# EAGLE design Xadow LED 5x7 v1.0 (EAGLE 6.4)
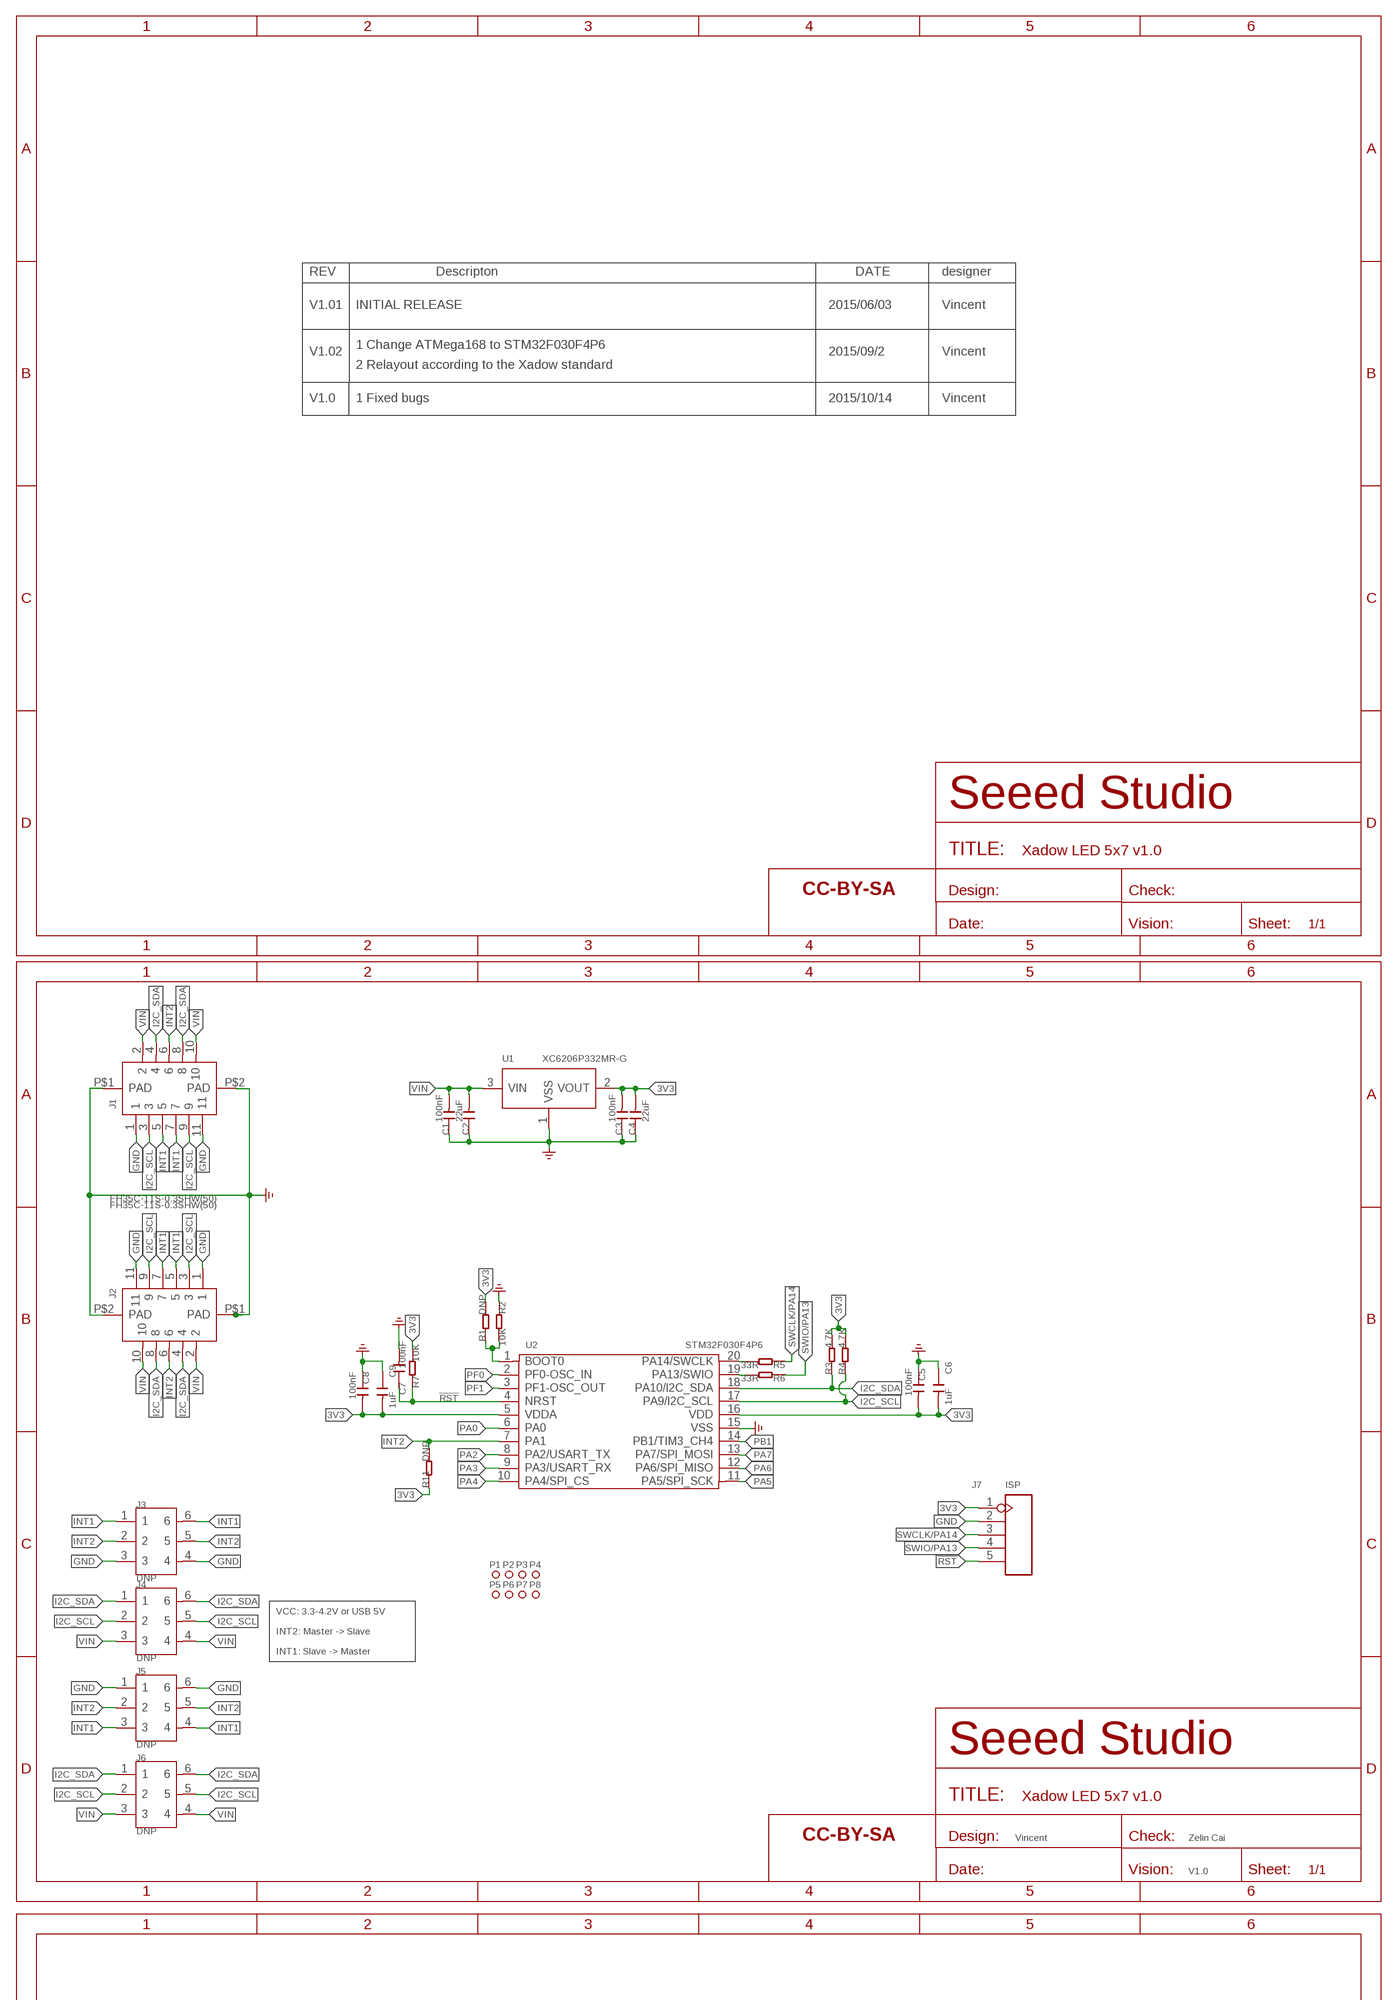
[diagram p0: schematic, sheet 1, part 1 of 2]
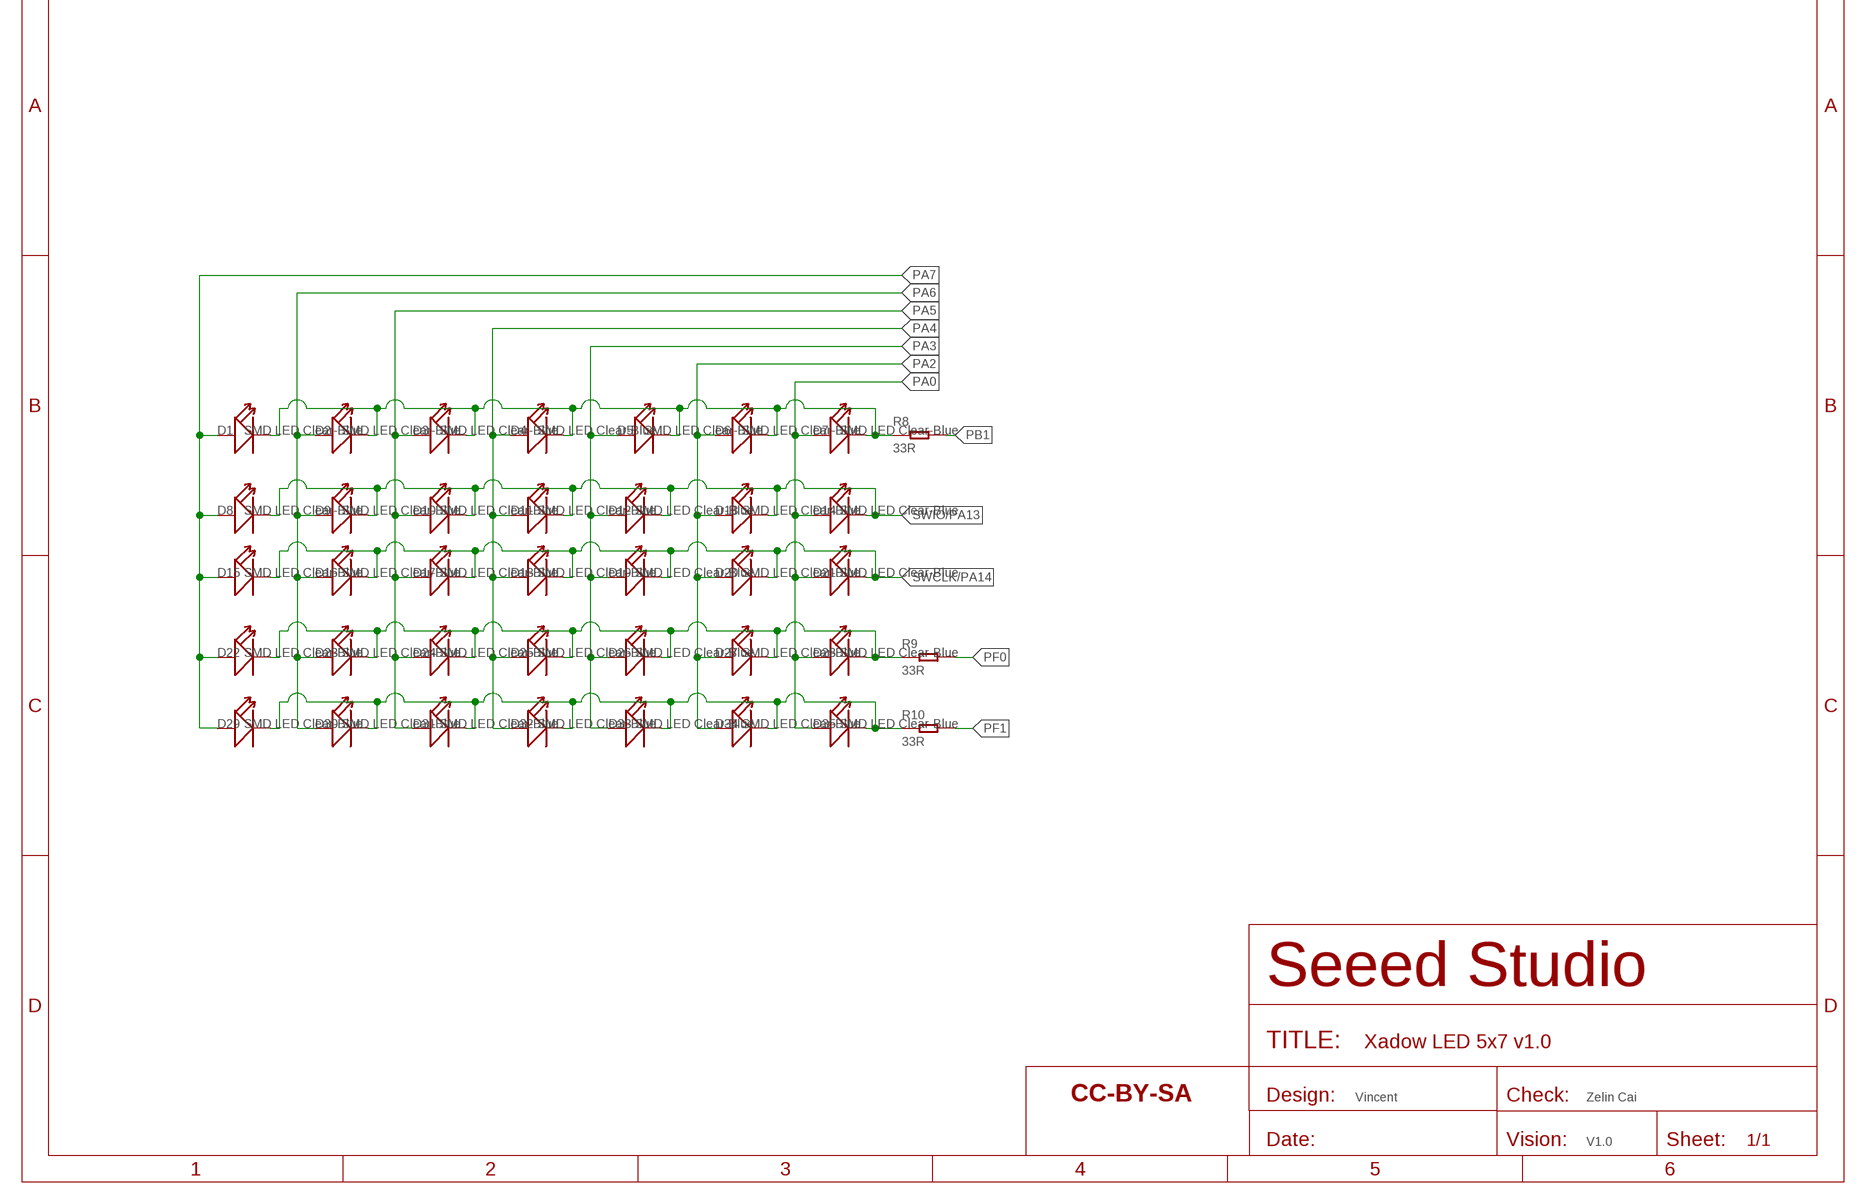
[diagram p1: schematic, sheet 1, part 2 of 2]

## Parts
C1  100nF  CAP-0402  [C0402]
C2  22uF  CAP-0603  [C0603]
C3  100nF  CAP-0402  [C0402]
C4  22uF  CAP-0603  [C0603]
C5  100nF  CAP-0402  [C0402]
C6  1uF  CAP-0402  [C0402]
C7  100nF  CAP-0402  [C0402]
C8  100nF  CAP-0402  [C0402]
C9  1uF  CAP-0402  [C0402]
D1  SMD LED Clear-Blue  LED'0603'  [LED-0603]
D2  SMD LED Clear-Blue  LED'0603'  [LED-0603]
D3  SMD LED Clear-Blue  LED'0603'  [LED-0603]
D4  SMD LED Clear-Blue  LED'0603'  [LED-0603]
D5  SMD LED Clear-Blue  LED'0603'  [LED-0603]
D6  SMD LED Clear-Blue  LED'0603'  [LED-0603]
D7  SMD LED Clear-Blue  LED'0603'  [LED-0603]
D8  SMD LED Clear-Blue  LED'0603'  [LED-0603]
D9  SMD LED Clear-Blue  LED'0603'  [LED-0603]
D10  SMD LED Clear-Blue  LED'0603'  [LED-0603]
D11  SMD LED Clear-Blue  LED'0603'  [LED-0603]
D12  SMD LED Clear-Blue  LED'0603'  [LED-0603]
D13  SMD LED Clear-Blue  LED'0603'  [LED-0603]
D14  SMD LED Clear-Blue  LED'0603'  [LED-0603]
D15  SMD LED Clear-Blue  LED'0603'  [LED-0603]
D16  SMD LED Clear-Blue  LED'0603'  [LED-0603]
D17  SMD LED Clear-Blue  LED'0603'  [LED-0603]
D18  SMD LED Clear-Blue  LED'0603'  [LED-0603]
D19  SMD LED Clear-Blue  LED'0603'  [LED-0603]
D20  SMD LED Clear-Blue  LED'0603'  [LED-0603]
D21  SMD LED Clear-Blue  LED'0603'  [LED-0603]
D22  SMD LED Clear-Blue  LED'0603'  [LED-0603]
D23  SMD LED Clear-Blue  LED'0603'  [LED-0603]
D24  SMD LED Clear-Blue  LED'0603'  [LED-0603]
D25  SMD LED Clear-Blue  LED'0603'  [LED-0603]
D26  SMD LED Clear-Blue  LED'0603'  [LED-0603]
D27  SMD LED Clear-Blue  LED'0603'  [LED-0603]
D28  SMD LED Clear-Blue  LED'0603'  [LED-0603]
D29  SMD LED Clear-Blue  LED'0603'  [LED-0603]
D30  SMD LED Clear-Blue  LED'0603'  [LED-0603]
D31  SMD LED Clear-Blue  LED'0603'  [LED-0603]
D32  SMD LED Clear-Blue  LED'0603'  [LED-0603]
D33  SMD LED Clear-Blue  LED'0603'  [LED-0603]
D34  SMD LED Clear-Blue  LED'0603'  [LED-0603]
D35  SMD LED Clear-Blue  LED'0603'  [LED-0603]
J1  FH35C-11S-0.3SHW(50)  FPC-CONNECTER-11P(FH35C-11S-0.3SHW(50))  [FPC11-SMD-0.3(FH35C)]
J2  FH35C-11S-0.3SHW(50)  FPC-CONNECTER-11P(FH35C-11S-0.3SHW(50))  [FPC11-SMD-0.3(FH35C)]
J3  DNP  HEADER6_ROUND  [6P-DIP-2_ROUND]
J4  DNP  HEADER6  [6P-DIP-2]
J5  DNP  HEADER6_ROUND  [6P-DIP-2_ROUND]
J6  DNP  HEADER6  [6P-DIP-2]
J7  ISP  HEADER-5PTEST  [H5-SMD-2.0-TEST]
P1  MARK-1.0'ANNULAR'  [ROUND-MARK-1.0]
P2  MARK-1.0'ANNULAR'  [ROUND-MARK-1.0]
P3  MARK-1.0'ANNULAR'  [ROUND-MARK-1.0]
P4  MARK-1.0'ANNULAR'  [ROUND-MARK-1.0]
P5  MARK-1.0'ANNULAR'  [ROUND-MARK-1.0]
P6  MARK-1.0'ANNULAR'  [ROUND-MARK-1.0]
P7  MARK-1.0'ANNULAR'  [ROUND-MARK-1.0]
P8  MARK-1.0'ANNULAR'  [ROUND-MARK-1.0]
R1  DNP  RES-0402  [R0402]
R2  10K  RES-0402  [R0402]
R3  4.7K  RES-0402  [R0402]
R4  4.7K  RES-0402  [R0402]
R5  33R  RES-0402  [R0402]
R6  33R  RES-0402  [R0402]
R7  10K  RES-0402  [R0402]
R8  33R  RES-0402  [R0402]
R9  33R  RES-0402  [R0402]
R10  33R  RES-0402  [R0402]
R11  DNP  RES-0402  [R0402]
U1  XC6206P332MR-G  PMIC-XC6206PMR  [SOT-23]
U2  STM32F030F4P6  MCU-STM32F030  [TSSOP20-0.65-6.5X4.4MM]
U$1  SEEEDSTUDIO-OPEN-SCH-FRAME  [SEEEDSTUDIO-PCB-FRAME]
U$2  SEEEDSTUDIO-OPEN-SCH-FRAME  [SEEEDSTUDIO-PCB-FRAME]
U$6  SEEEDSTUDIO-OPEN-SCH-FRAME  [SEEEDSTUDIO-PCB-FRAME]

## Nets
3V3: C3.2 C4.2 C5.2 C6.2 C8.2 C9.2 J7.1 R1.2 R3.2 R4.2 R7.2 R11.1 U1.2(VOUT) U2.5(VDDA) U2.16(VDD)
!RST: C7.1 J7.5 R7.1 U2.4(NRST)
GND: C1.1 C2.1 C3.1 C4.1 C5.1 C6.1 C7.2 C8.1 C9.1 J1.1 J1.11 J1.P$1(PAD) J1.P$2(PAD) J2.1 J2.11 J2.P$1(PAD) J2.P$2(PAD) J3.3 J3.4 J5.1 J5.6 J7.2 R2.1 U1.1(VSS) U2.15(VSS) ; supply symbol labelled GND_POWER
I2C_SCL: J1.3 J1.9 J2.3 J2.9 J4.2 J4.5 J6.2 J6.5 R4.1 U2.17(PA9/I2C_SCL)
I2C_SDA: J1.4 J1.8 J2.4 J2.8 J4.1 J4.6 J6.1 J6.6 R3.1 U2.18(PA10/I2C_SDA)
INT1: J1.5 J1.7 J2.5 J2.7 J3.1 J3.6 J5.3 J5.4
INT2: J1.6 J2.6 J3.2 J3.5 J5.2 J5.5 R11.2 U2.7(PA1)
N$3: D29.- D30.- D31.- D32.- D33.- D34.- D35.- R10.1
N$4: D22.- D23.- D24.- D25.- D26.- D27.- D28.- R9.1
N$5: D1.- D2.- D3.- D4.- D5.- D6.- D7.- R8.1
N$6: R1.1 R2.2 U2.1(BOOT0)
N$7: R5.2 U2.20(PA14/SWCLK)
N$8: R6.2 U2.19(PA13/SWIO)
PA0: D7.+ D14.+ D21.+ D28.+ D35.+ U2.6(PA0)
PA2: D6.+ D13.+ D20.+ D27.+ D34.+ U2.8(PA2/USART_TX)
PA3: D5.+ D12.+ D19.+ D26.+ D33.+ U2.9(PA3/USART_RX)
PA4: D4.+ D11.+ D18.+ D25.+ D32.+ U2.10(PA4/SPI_CS)
PA5: D3.+ D10.+ D17.+ D24.+ D31.+ U2.11(PA5/SPI_SCK)
PA6: D2.+ D9.+ D16.+ D23.+ D30.+ U2.12(PA6/SPI_MISO)
PA7: D1.+ D8.+ D15.+ D22.+ D29.+ U2.13(PA7/SPI_MOSI)
PB1: R8.2 U2.14(PB1/TIM3_CH4)
PF0: R9.2 U2.2(PF0-OSC_IN)
PF1: R10.2 U2.3(PF1-OSC_OUT)
SWCLK/PA14: D15.- D16.- D17.- D18.- D19.- D20.- D21.- J7.3 R5.1
SWIO/PA13: D8.- D9.- D10.- D11.- D12.- D13.- D14.- J7.4 R6.1
VIN: C1.2 C2.2 J1.2 J1.10 J2.2 J2.10 J4.3 J4.4 J6.3 J6.4 U1.3(VIN)

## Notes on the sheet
- REV | Descripton | DATE | designer
- V1.01 | INITIAL RELEASE | 2015/06/03 | Vincent
- 1 Change ATMega168 to STM32F030F4P6
- V1.02 | 2015/09/2 | Vincent
- 2 Relayout according to the Xadow standard
- V1.0 | 1 Fixed bugs | 2015/10/14 | Vincent
- VCC: 3.3-4.2V or USB 5V
- INT2: Master -> Slave
- INT1: Slave -> Master
- Vincent | Zelin Cai
- V1.0
- Vincent | Zelin Cai
- V1.0

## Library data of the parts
C1-C9 = Discrete-new:CAP: Ceramic Capacitors
D1-D35 = Discrete:LED*
J1 J2 = template:FPC-CONNECTER-11P(FH35C-11S-0.3SHW(50))
J3 J5 = template:HEADER6_ROUND
J4 J6 = template:HEADER6
J7 = Connector-new:HEADER-5P
P1-P8 = Discrete-new:MARK-1.0; PARTNO: DNP
R1-R11 = Discrete-new:RES
U1 = IC-new:PMIC-XC6206P: LOW ESR Cap.Compatible Positive Voltage Regulators
U2 = IC-new:MCU-STM32F030
U$1 U$2 U$6 = moudle-new:SEEEDSTUDIO-OPEN-SCH-FRAME

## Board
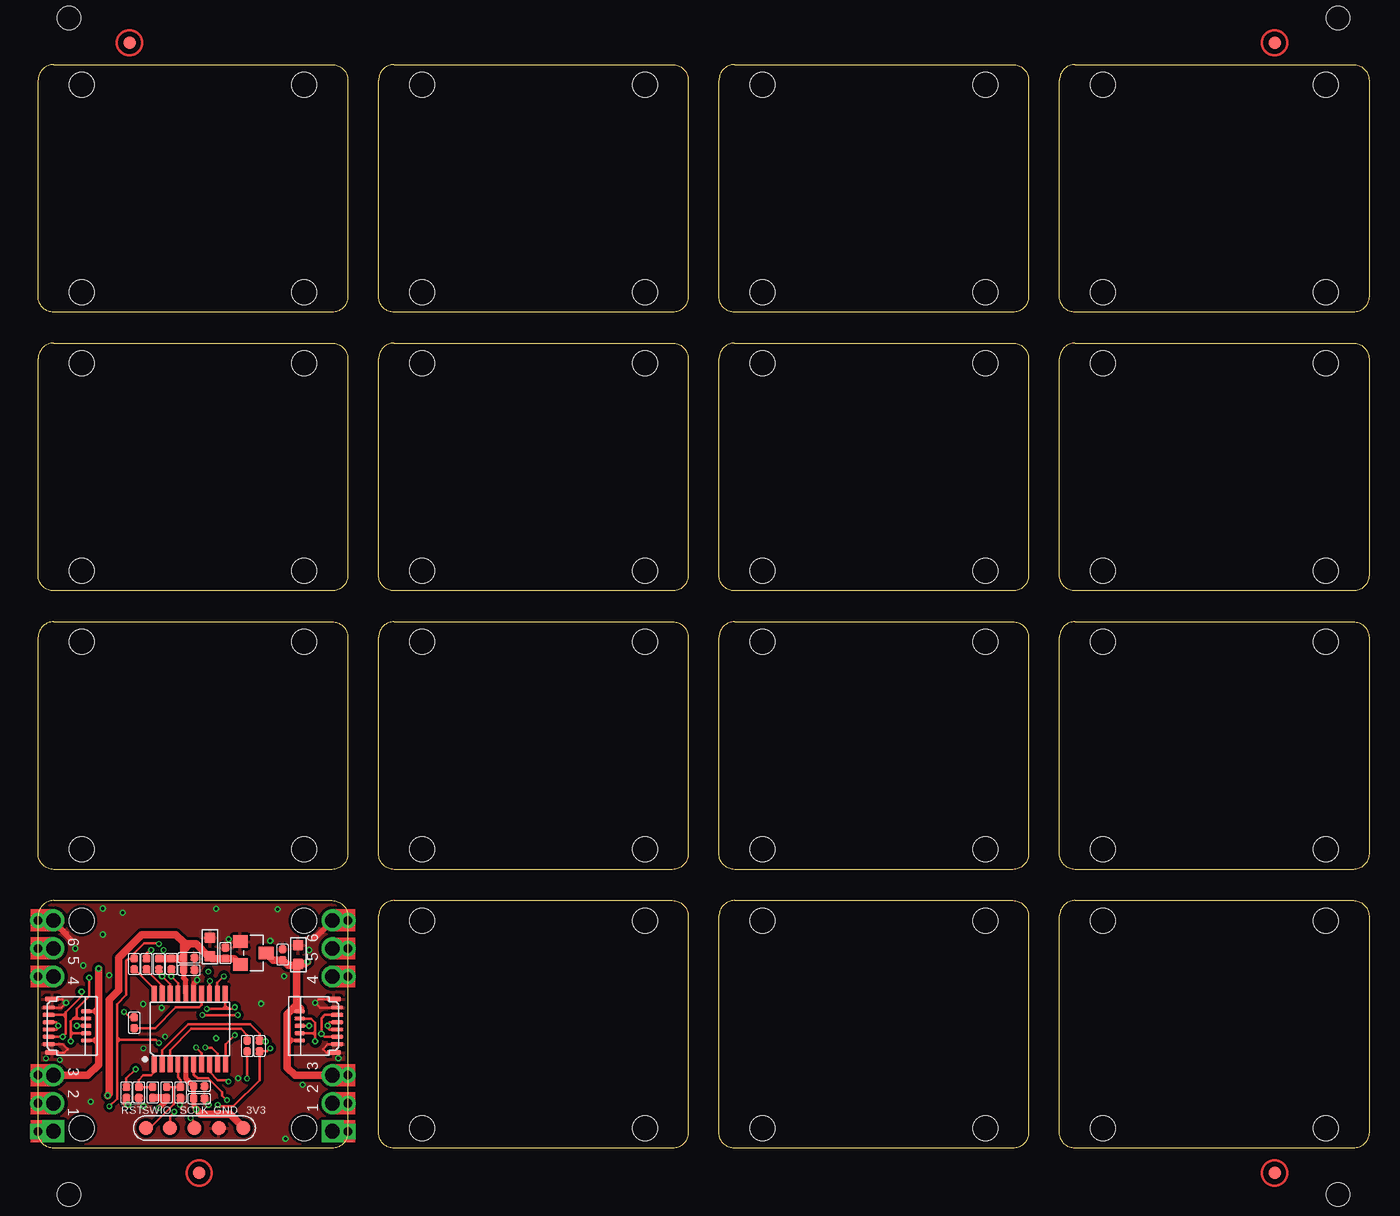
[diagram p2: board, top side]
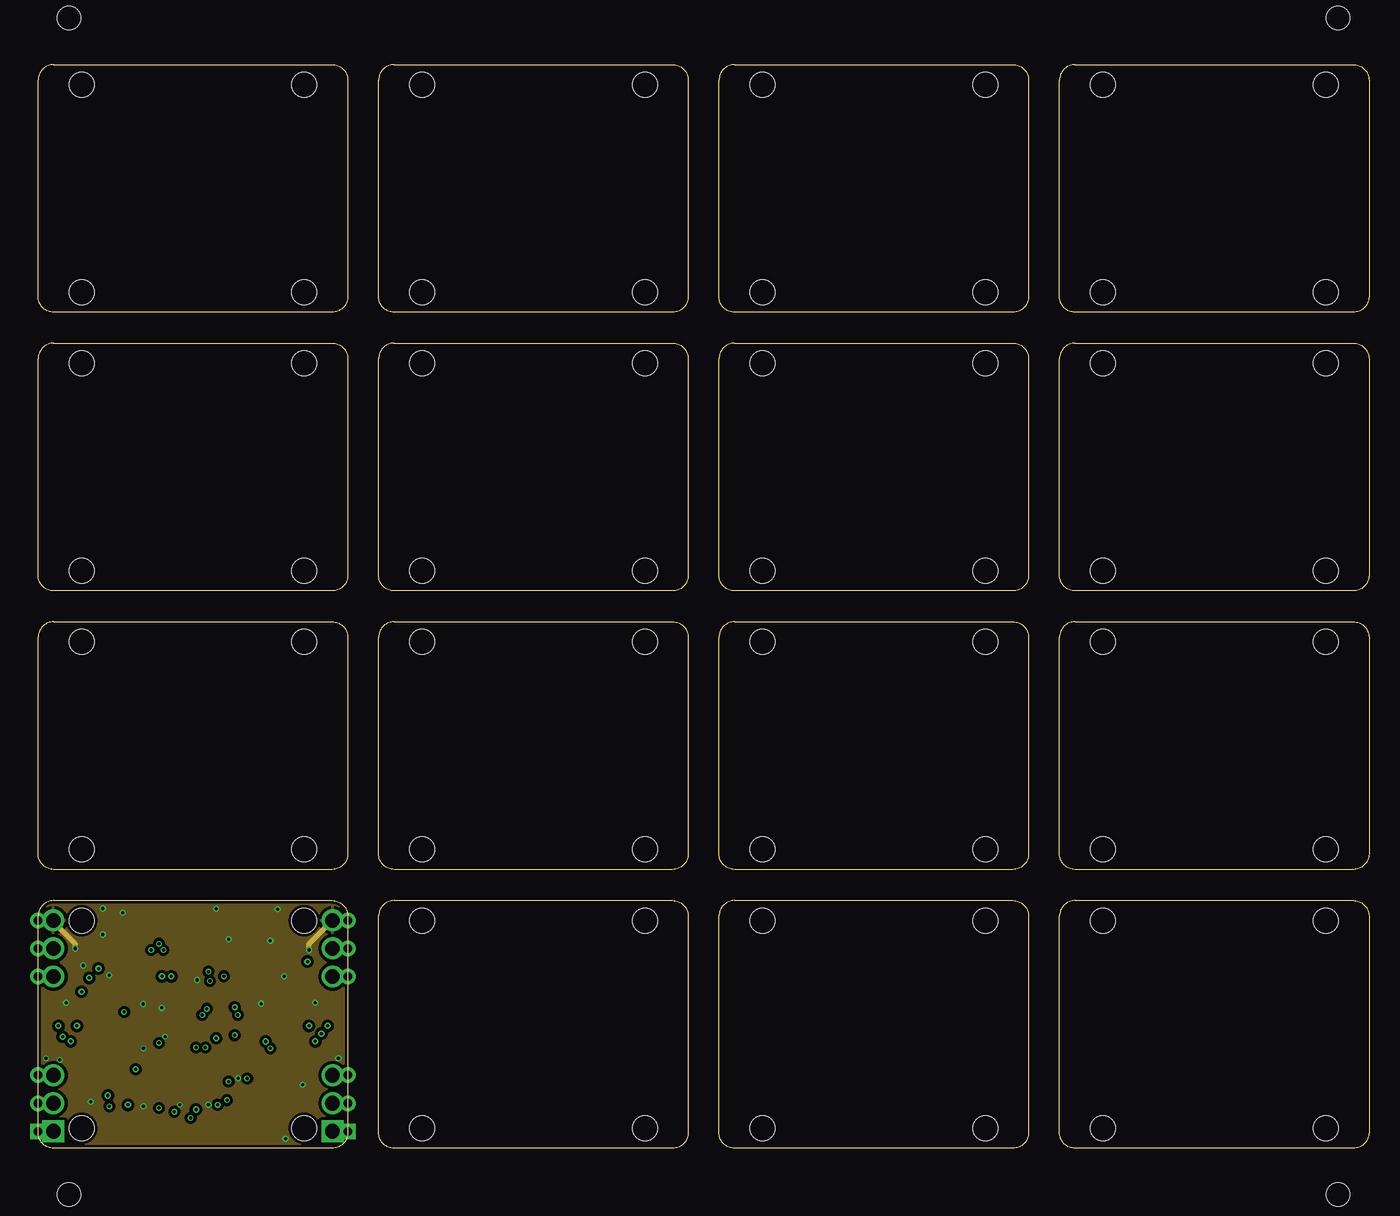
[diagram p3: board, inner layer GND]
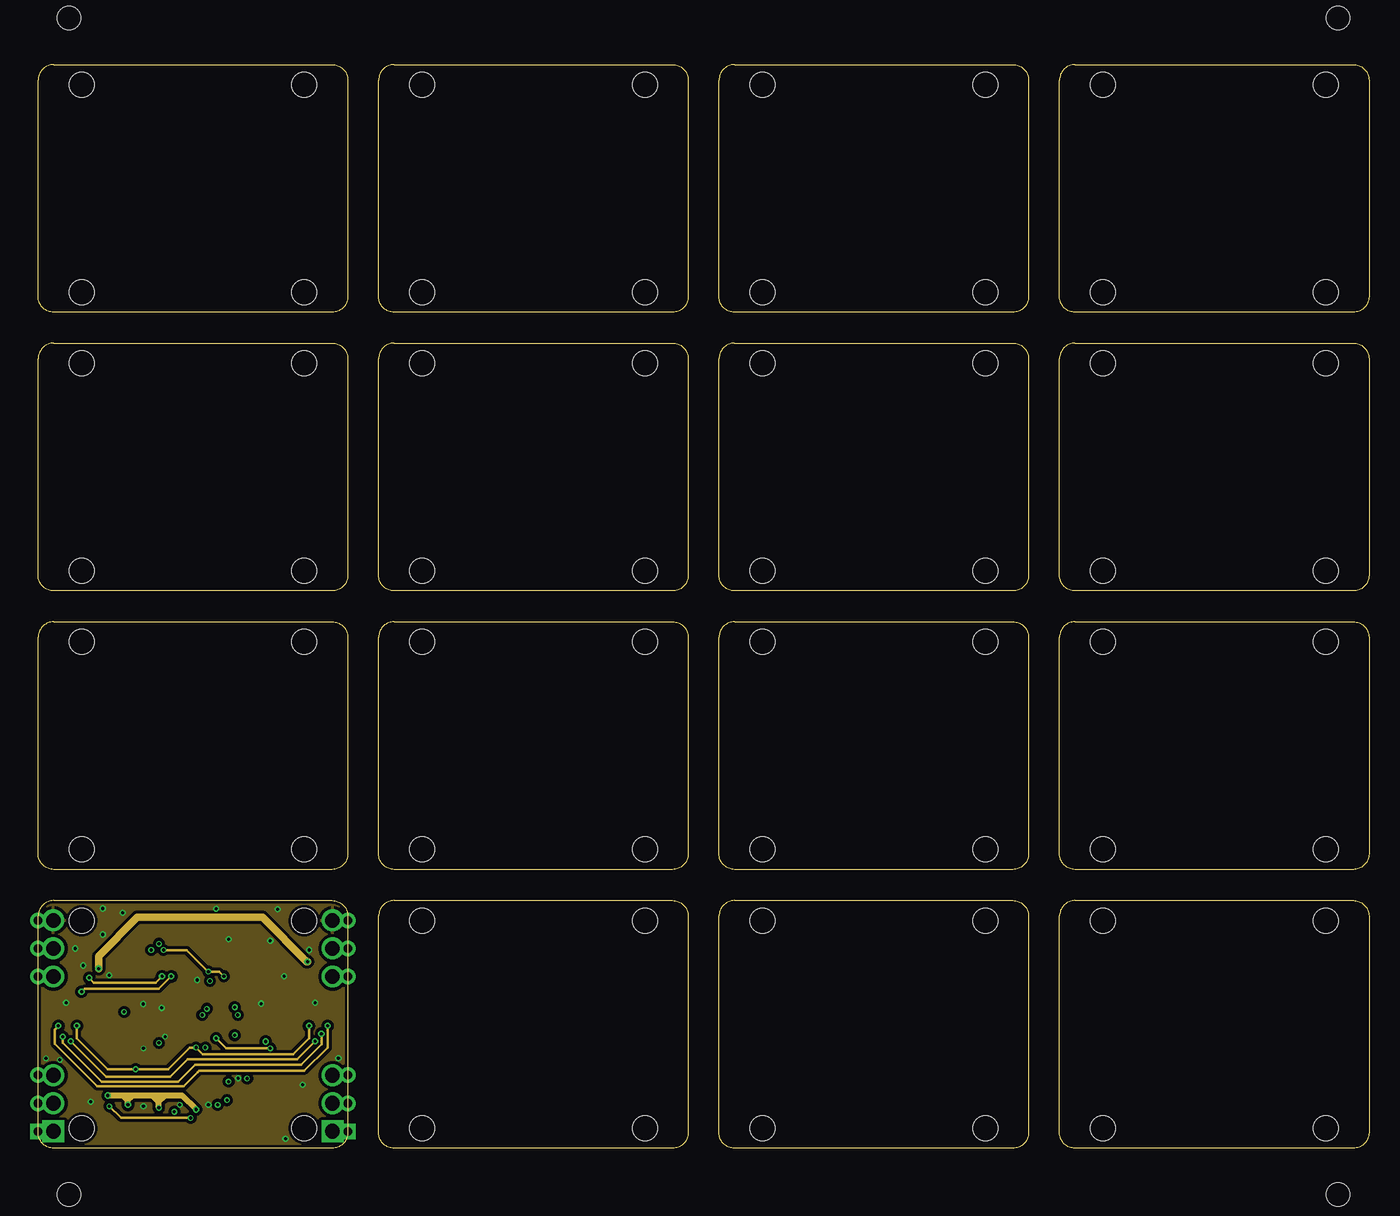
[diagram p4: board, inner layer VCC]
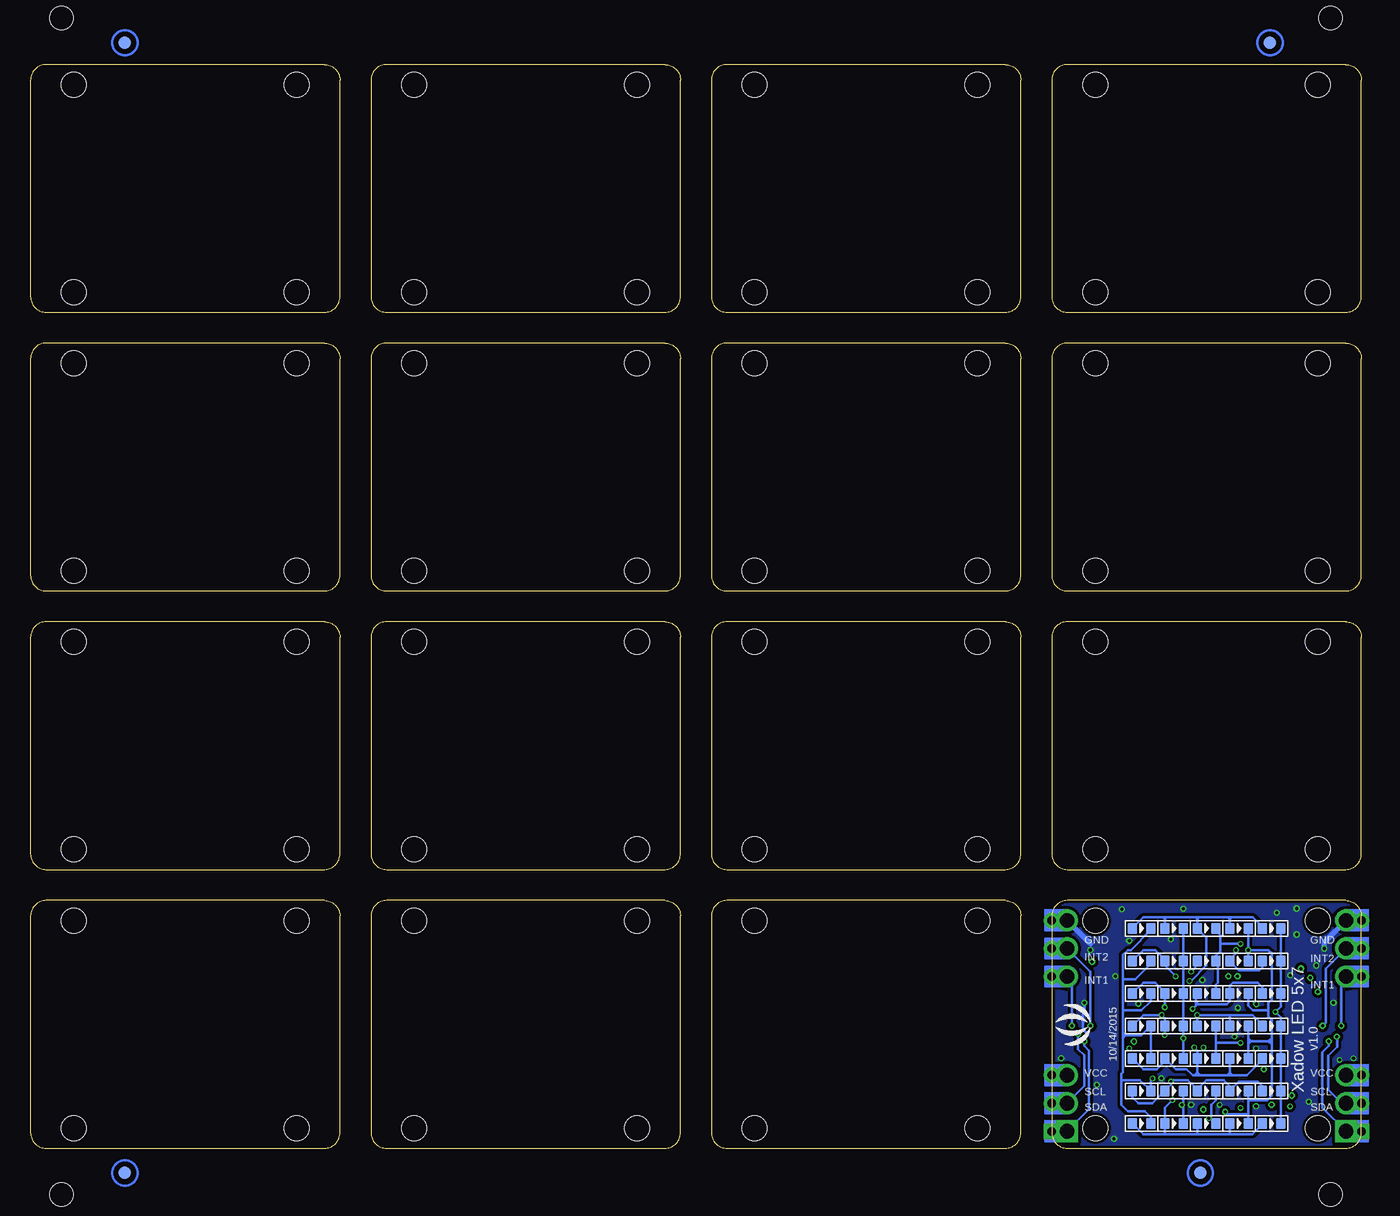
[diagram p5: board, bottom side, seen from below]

Size 109.22 x 88.9 mm. Coordinates in mm from the lower left corner, seen from the top.
Outline: 181 segments
Copper layers (1*2*15*16): Top 0.035mm / dielectric 0.2mm / GND 0.0175mm / dielectric 0.3mm / VCC 0.0175mm / dielectric 0.2mm / Bottom 0.035mm
Design rules "SeeedStudio_4layer_DRU_no_angle_20140221 *": minimum track width 8mil, minimum drill 10mil, track to track 6mil, track to pad 6mil, pad to pad 6mil, via to via 6mil, smd to smd 0mil, copper to edge 10mil, drill to drill 8mil, minimum pad ring 6mil, minimum via ring 4mil, stop-mask expansion 4mil, vias tented up to drill 100mil, thermal gap 10mil
Holes 2.03 mm at 21.84,1.65 21.84,18.67 3.56,18.67 3.56,1.65 3.56,1.65 3.56,18.67 21.84,18.67 21.84,1.65 49.78,1.65 49.78,18.67 31.5,18.67 31.5,1.65 21.84,24.51 21.84,41.53 3.56,41.53 3.56,24.51 49.78,24.51 49.78,41.53 31.5,41.53 31.5,24.51 77.72,1.65 77.72,18.67 59.44,18.67 59.44,1.65 105.66,1.65 105.66,18.67 87.38,18.67 87.38,1.65 77.72,24.51 77.72,41.53 59.44,41.53 59.44,24.51 105.66,24.51 105.66,41.53 87.38,41.53 87.38,24.51 21.84,47.37 21.84,64.39 3.56,64.39 3.56,47.37 49.78,47.37 49.78,64.39 31.5,64.39 31.5,47.37 21.84,70.23 21.84,87.25 3.56,87.25 3.56,70.23 49.78,70.23 49.78,87.25 31.5,87.25 31.5,70.23 77.72,47.37 77.72,64.39 59.44,64.39 59.44,47.37 105.66,47.37 105.66,64.39 87.38,64.39 87.38,47.37 77.72,70.23 77.72,87.25 59.44,87.25 59.44,70.23 105.66,70.23 105.66,87.25 87.38,87.25 87.38,70.23
Holes 1.91 mm at 2.54,-3.81 106.68,-3.81 106.68,92.71 2.54,92.71

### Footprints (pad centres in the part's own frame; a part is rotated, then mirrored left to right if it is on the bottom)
C0402 = smd 0.635 x 0.635: 1 0,0.445; 2 0,-0.445
C0603 = smd 0.889 x 0.889: 1 0,0.762; 2 0,-0.762
LED-0603 = smd 0.762 x 0.889: + -0.762,0; - 0.762,0
FPC11-SMD-0.3(FH35C) = smd 0.3 x 1: 1 -1.5,-3.075; 3 -0.9,-3.075; 5 -0.3,-3.075; 7 0.3,-3.075; 9 0.9,-3.075; 11 1.5,-3.075 | smd 0.3 x 0.85: 2 -1.2,0; 4 -0.6,0; 6 0,0; 8 0.6,0; 10 1.2,0 | smd 0.4 x 1.15: P$1 2.2,-2.8; P$2 -2.2,-2.8
6P-DIP-2_ROUND = drill 0.7 pad 1.27: 1 -2.3,0; 2 0,0; 3 2.3,0 | drill 1.2 pad 1.8: 4 2.3,1.25; 5 0,1.25; 6 -2.3,1.25
6P-DIP-2 = drill 0.7 pad 1.27 square: 1 -2.3,0 | drill 0.7 pad 1.27: 2 0,0; 3 2.3,0 | drill 1.2 pad 1.8: 4 2.3,1.25; 5 0,1.25 | drill 1.2 pad 1.8 square: 6 -2.3,1.25
H5-SMD-2.0-TEST = smd 1.143 x 1.143: 1 0,4; 2 0,2; 3 0,0; 4 0,-2; 5 0,-4
ROUND-MARK-1.0 = smd 1.016 x 1.016: P$1 0,0
R0402 = smd 0.635 x 0.635: 1 0,0.445; 2 0,-0.445
SOT-23 = smd 1.016 x 1.2: 1 -0.95,-1.06; 2 0.95,-1.06; 3 0,1.06
TSSOP20-0.65-6.5X4.4MM = smd 0.4 x 1.35: 1 -2.925,-2.875; 2 -2.275,-2.875; 3 -1.625,-2.875; 4 -0.975,-2.875; 5 -0.325,-2.875; 6 0.325,-2.875; 7 0.975,-2.875; 8 1.625,-2.875; 9 2.275,-2.875; 10 2.925,-2.875; 11 2.91,2.875; 12 2.26,2.875; 13 1.61,2.875; 14 0.96,2.875; 15 0.325,2.875; 16 -0.325,2.875; 17 -0.975,2.875; 18 -1.625,2.875; 19 -2.275,2.875; 20 -2.925,2.875

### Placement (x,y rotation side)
C1  20.07,15.88 0 top
C2  21.34,15.88 0 top
C3  15.37,16 0 top
C4  14.1,16.51 0 top
C5  12.38,14.61 270 top
C6  12.38,15.62 270 top
C7  11.68,4.57 0 top
C8  13.21,5.08 270 top
C9  13.21,4.06 270 top
D1  7.37,18.03 0 bottom
D2  7.37,15.37 0 bottom
D3  7.37,12.7 0 bottom
D4  7.37,10.03 0 bottom
D5  7.37,7.37 0 bottom
D6  7.37,4.7 0 bottom
D7  7.37,2.03 0 bottom
D8  10.03,18.03 0 bottom
D9  10.03,15.37 0 bottom
D10  10.03,12.7 0 bottom
D11  10.03,10.03 0 bottom
D12  10.03,7.37 0 bottom
D13  10.03,4.7 0 bottom
D14  10.03,2.03 0 bottom
D15  12.7,18.03 0 bottom
D16  12.7,15.37 0 bottom
D17  12.7,12.7 0 bottom
D18  12.7,10.03 0 bottom
D19  12.7,7.37 0 bottom
D20  12.7,4.7 0 bottom
D21  12.7,2.03 0 bottom
D22  15.37,18.03 0 bottom
D23  15.37,15.37 0 bottom
D24  15.37,12.7 0 bottom
D25  15.37,10.03 0 bottom
D26  15.37,7.37 0 bottom
D27  15.37,4.7 0 bottom
D28  15.37,2.03 0 bottom
D29  18.03,18.03 0 bottom
D30  18.03,15.37 0 bottom
D31  18.03,12.7 0 bottom
D32  18.03,10.03 0 bottom
D33  18.03,7.37 0 bottom
D34  18.03,4.7 0 bottom
D35  18.03,2.03 0 bottom
J1  3.94,10.03 270 top
J2  21.46,10.03 90 top
J3  25.4,16.38 90 top
J4  25.4,3.68 90 top
J5  0,16.38 270 top
J6  0,3.68 90 bottom
J7  12.83,1.65 270 top
P1  13.21,-2.03 90 top
P2  13.21,-2.03 270 bottom
P3  101.47,-2.03 90 top
P4  101.47,-2.03 270 bottom
P5  7.49,90.68 90 top
P6  7.49,90.68 270 bottom
P7  101.47,90.68 90 top
P8  101.47,90.68 270 bottom
R1  9.4,4.57 0 top
R2  8.25,4.57 180 top
R3  9.91,15.11 180 top
R4  10.92,15.11 180 top
R5  7.87,15.11 0 top
R6  8.89,15.11 0 top
R7  10.54,4.57 0 top
R8  7.87,10.29 0 top
R9  18.16,8.38 180 top
R10  17.14,8.38 180 top
R11  7.24,4.57 180 top
U1  17.65,16 270 top
U2  12.45,9.78 0 top
U$1  not placed on the board
U$2  not placed on the board
U$4  [SEEED-SILK-160*153MIL]  23.75,10.16 90 bottom
U$6  not placed on the board

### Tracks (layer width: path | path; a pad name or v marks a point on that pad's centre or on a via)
3V3  (via drill 0.25, 0.25 pad 0.51)
  Top 0.406: U2.5 12.12,5.72 C8.2 C9.2 12.76,3.36 v12.95,3.17 | C5.2 11.94,13.97 12.12,13.79 U2.16
  Top 0.508: R7.2 10.54,3.94 v9.91,3.3
  Top 0.61: R1.2 R7.2 | R3.2 R4.2 11.87,15.56 11.94,15.49 | C5.2 11.94,15.49 | 11.94,15.49 C6.2 11.94,16.26 | J7.1 16.83,1.71 15.75,2.79 13.34,2.79 v12.95,3.17 | v5.71,4.32 5.84,4.44 5.84,12.19 6.6,12.95 6.6,15.62 8.51,17.53 11.3,17.53 11.94,16.89 | R11.1 7.24,3.68 v7.37,3.56 | 12.45,16.76 12.95,16.76 13.97,15.75 C4.2 14.29,15.56 C3.2 16.09,15.56 U1.2 | 12.45,16.76 12.06,16.76 11.94,16.89 | 11.94,16.26 11.94,16.89 | 12.45,16.76 11.94,16.26
  VCC 0.508: v12.95,3.17 11.81,4.32 10.41,4.32 | 10.41,4.32 9.91,4.32 | 9.91,4.32 9.4,4.32 | 9.4,4.32 7.75,4.32 | 7.75,4.32 7.37,4.32 | 7.37,4.32 6.98,4.32 | 6.98,4.32 v5.71,4.32 | v9.91,3.3 9.91,3.81 | 9.91,3.81 9.91,4.32 | 9.4,4.32 9.91,3.81 | 9.91,3.81 10.41,4.32 | v7.37,3.56 7.37,3.94 | 7.37,3.94 7.37,4.32 | 6.98,4.32 7.37,3.94 | 7.37,3.94 7.75,4.32
!RST
  Top 0.203: U2.4 11.47,5.8 11.68,5.59 C7.1 11.24,5.02 | R7.1 10.99,5.02 | 10.99,5.02 11.11,5.02 | 11.11,5.02 11.24,5.02 | J7.5 9.14,1.65 11.11,3.62 11.11,4.76 11.11,4.89 | 11.11,4.89 11.11,5.02 | 11.11,4.89 10.99,5.02 | 11.11,4.89 11.24,5.02
GND  (via drill 0.25, 0.25 pad 0.51)
  Top 0.203: J5.6 1.38,18.68 2.41,17.65 | J3.4 24.15,18.43 23.37,17.65 | 23.66,12.23 J2.P$1 23.03,12.23 v22.73,11.94 23.14,11.53 J2.11 | J2.1 23.77,8.53 23.37,8.13 23.66,7.83 J2.P$2 24.3,7.87 24.64,7.87 v24.64,7.37 | J1.1 1.88,11.53 v2.29,11.94 1.99,12.23 J1.P$2 | J1.11 2.01,8.53 2.41,8.13 2.12,7.83 J1.P$1
  Top 0.406: J3.4 22.61,17.14 | 1.14,18.67 2.67,17.14 | U2.15 12.77,13.51 v13.06,13.79 | 11.68,3.81 11.68,3.56 v11.62,3.56 | C9.1 13.65,3.87 v13.97,3.56
  Top 0.508: C7.2 11.68,3.81
  GND 0.406: v22.23,16.26 22.23,16.76 24.13,18.67 | v3.05,16.38 3.05,16.76 1.14,18.67
  Bottom 0.203: v22.73,11.94 22.73,11.18 22.86,11.05 22.86,9.78 22.61,9.52
  Bottom 0.406: v3.05,16.38 3.05,16.88 J5.6 | 22.23,16.76 J3.4
  other vias: 5.82,14.17 4.32,3.81 3.68,14.99 5.31,19.66 19.05,17.02 14.61,19.65 20.19,14.1 18.29,11.86 8.64,3.43 19.66,19.61 20.29,0.76 6.93,19.3 15.62,17.14 21.69,5.21 10.13,11.51 8.61,11.82 16.41,5.73 8.64,8.19 1.78,7.24 0.63,7.37 10.41,9.14 5.31,17.53
  pour Top (isolate 0.254): -0.76,-0.13 26.54,-0.13 26.54,20.83 -0.76,20.83
  pour Bottom (isolate 0.254): -0.76,-0.13 26.54,-0.13 26.54,20.83 -0.76,20.83
  pour VCC (isolate 0.254, rank 6): 0,0 25.4,0 25.27,20.32 0,20.32
  pour GND (isolate 0.254): 0,0 25.4,0 25.27,20.32 0,20.32
I2C_SCL  (via drill 0.25 pad 0.51)
  Top 0.203: J2.9 23.51,10.93 23.24,10.67 v23.24,9.4 23.51,9.13 J2.3 | J1.3 2.02,10.93 | 2.04,10.93 2.25,10.93 2.26,10.92 | J1.9 v2,9.13 v2.01,9.14 2.26,9.4 2.26,10.92 | 2.26,11.15 2.26,10.92 | 2.26,11.15 3.56,12.45 v3.56,12.83 | 2.02,10.93 2.04,10.93 | 2.04,10.93 2.26,11.15 | 2.02,10.93 2.22,10.73 | R4.1 v10.92,14.1 11.47,13.55 U2.17
  VCC 0.203: v23.24,9.4 23.24,8.51 21.59,6.86 12.87,6.86 11.47,5.46 5.21,5.46 2.01,8.66 v2.01,9.14 | v10.92,14.1 9.91,13.08 3.81,13.08 v3.56,12.83
  Bottom 0.203: J4.2 J4.5 22.73,5.1 22.73,7.62 23.24,8.13 v23.24,9.4 | J6.2 J6.5 | J6.5 1.61,3.69 2.72,4.8 2.72,7.57 1.98,8.31 1.98,9.12 v2.01,9.14
  Bottom 0.254: J6.5
I2C_SDA  (via drill 0.25 pad 0.51)
  Top 0.203: 21.43,9.4 J2.4 22.51,9.43 | J2.8 22.39,10.63 22.73,10.29 22.73,9.65 | 22.73,9.65 22.73,9.4 | 22.73,9.4 22.73,9.21 | 22.73,9.21 v22.73,8.76 | 22.51,9.43 22.7,9.43 22.73,9.4 | J1.8 2.89,9.43 | 2.89,9.43 2.7,9.43 2.67,9.4 | 2.67,9.65 2.67,10.41 2.89,10.63 3.17,10.63 | 2.67,9.65 2.67,9.4 | 2.67,9.4 2.67,9.21 | 2.67,9.21 v2.67,8.76 | 22.51,9.43 | 22.51,9.43 22.73,9.65 | 22.51,9.43 22.73,9.21 | 2.89,9.43 | 2.89,9.43 2.67,9.65 | 2.89,9.43 2.67,9.21 | 3.17,10.63 3.17,10.79 | J1.4 3.17,10.63 | 3.17,10.92 2.92,10.67 | 3.17,10.92 3.17,10.79 | 3.17,10.79 3.3,10.67 | U2.18 10.82,13.44 v10.16,14.1 9.91,14.35 R3.1 | 3.17,10.92 3.17,11.43 4.19,12.45 v4.19,13.97
  Top 0.406: J4.6 J4.1
  VCC 0.203: v22.73,8.76 21.26,7.29 12.28,7.29 10.83,5.84 5.59,5.84 v2.67,8.76 | v10.16,14.1 9.65,13.59 4.57,13.59 v4.19,13.97
  Bottom 0.203: J4.6 22.35,3.18 22.35,8 22.73,8.38 v22.73,8.76 | v2.67,8.76 2.67,8.38 3.2,7.85 3.2,3.33 J6.6 | J6.6 J6.1 | J6.6 1.25,1.45
INT1  (via drill 0.25 pad 0.51)
  Top 0.203: J2.5 23.92,9.73 23.75,9.91 v23.75,10.03 23.75,10.16 23.92,10.33 J2.7 | J1.7 1.48,9.73 1.65,9.91 v1.65,10.03 1.65,10.16 1.48,10.33 J1.5
  Top 0.406: J3.6 J3.1
  VCC 0.203: v23.75,10.03 23.75,8.25 21.84,6.35 13.21,6.35 13.08,6.22 11.94,5.08 4.83,5.08 1.35,8.56 1.35,9.73 v1.65,10.03
  Bottom 0.203: v1.65,10.03 1.65,13.68 J5.4 J5.3 | v23.75,10.03 23.75,13.68 J3.6
INT2  (via drill 0.25, 0.25 pad 0.51)
  Top 0.203: J2.6 v22.23,10.03 | J1.6 v3.17,10.03 | U2.7 13.42,7.79 v12.95,8.25 | R11.2 7.24,5.72 v8,6.48
  VCC 0.203: v3.17,10.03 3.17,9.02 5.71,6.48 v8,6.48 10.67,6.48 12.45,8.25 v12.95,8.25 13.51,7.7 20.9,7.7 22.23,9.02 v22.23,10.03
  Bottom 0.203: J5.2 J5.5 2.92,14.71 2.92,10.29 v3.17,10.03 | v22.23,10.03 22.23,14.46 J3.5 J3.2
N$3  (via drill 0.25)
  Top 0.203: R10.1 v17.14,5.72
  Bottom 0.203: D35.- 17.27,2.54 17.78,3.05 19.18,3.05 19.69,3.56 19.69,5.59 | 19.69,5.59 19.69,6.1 19.56,6.22 19.56,9.02 | D29.- 17.27,17.91 18.92,16.26 19.18,16.26 19.56,15.88 19.56,13.84 | 19.56,13.84 19.56,11.3 | 19.56,11.3 19.56,9.52 | 19.56,9.52 19.56,9.27 | 19.56,9.27 19.56,9.02 | D31.- 17.27,12.06 18.03,11.3 19.56,11.3 | D30.- 17.27,15.11 18.54,13.84 19.56,13.84 | 19.69,5.59 18.16,5.59 D34.- 17.27,5.59 v17.14,5.72 | 19.3,9.27 18.03,9.27 D32.- D33.- | 19.3,9.27 19.56,9.27 | 19.3,9.27 19.56,9.52 | 19.3,9.27 19.56,9.02
N$4  (via drill 0.25)
  Top 0.203: v19.05,8.19 18.8,7.94 R9.1 18.16,5.59 16,3.43 14.86,3.43 v14.73,3.56
  VCC 0.203: v19.05,8.19 15.43,8.19 v14.61,9.02
  Bottom 0.203: D22.- D23.- D24.- D25.- | D25.- v14.61,9.02 D26.- | 14.48,9.91 D25.- | D28.- 14.61,3.43 v14.73,3.56 14.61,3.68 D27.-
N$5  (via drill 0.25)
  Top 0.203: R8.1 7.49,10.73 v7.05,11.18
  Bottom 0.203: D1.- D2.- D3.- 6.6,11.62 v7.05,11.18 6.6,10.73 D4.- D5.- D6.- D7.-
N$6
  Top 0.203: U2.1 9.52,6.22 9.27,5.97 8.64,5.97 8.25,5.59 R2.2 R1.1
N$7
  Top 0.203: U2.20 9.52,13.09 7.94,14.67 R5.2
N$8
  Top 0.203: U2.19 10.17,13.32 8.89,14.61 R6.2
PA0  (via drill 0.25)
  Top 0.203: U2.6 12.77,6.02 13.08,5.72 13.97,5.72 15.11,4.57 15.11,4.32 v15.49,3.94
  Bottom 0.203: D7.+ 8.13,1.97 8.95,1.14 10.67,1.14 | 10.67,1.14 10.73,1.14 | 10.73,1.14 10.92,1.14 | 10.92,1.14 13.34,1.14 | 13.34,1.14 13.53,1.14 | 13.53,1.14 13.59,1.14 | 13.59,1.14 16,1.14 | 16,1.14 16.07,1.14 | 16.07,1.14 16.26,1.14 | 16.26,1.14 17.91,1.14 D35.+ | 16.13,1.27 D28.+ 16.13,3.3 v15.49,3.94 | 16.13,1.27 16.13,1.21 16.07,1.14 | D21.+ 13.46,1.27 | 13.46,1.27 13.46,1.21 13.53,1.14 | D14.+ 10.79,1.27 | 10.79,1.27 10.79,1.21 10.73,1.14 | 10.67,1.14 10.79,1.27 | 10.79,1.27 10.92,1.14 | 13.34,1.14 13.46,1.27 | 13.46,1.27 13.59,1.14 | 16,1.14 16.13,1.27 | 16.13,1.27 16.26,1.14
PA2  (via drill 0.25)
  Top 0.203: U2.8 14.07,6.25 14.73,5.59 15.49,5.59 v15.62,5.46
  Bottom 0.203: D34.+ 18.8,4.19 18.29,3.68 17.14,3.68 D27.+ 15.62,5.21 v15.62,5.46 15.49,5.59 14.22,5.59 13.46,4.83 | D6.+ 8.13,5.08 8.51,5.46 10.03,5.46 D13.+ 10.79,5.08 11.3,5.59 12.7,5.59 13.46,4.83 | D20.+ 13.46,4.83
PA3  (via drill 0.25)
  Top 0.203: U2.9 14.72,7.76 14.22,8.25 v13.72,8.25
  Bottom 0.203: D5.+ 8.13,7.24 9.4,5.97 10.54,5.97 | 10.54,5.97 10.79,5.97 | 10.79,5.97 11.05,5.97 | 11.05,5.97 13.21,5.97 | 13.21,5.97 13.46,5.97 | 13.46,5.97 13.72,5.97 | D12.+ 10.79,6.22 | 10.79,6.22 10.79,5.97 | 13.46,6.22 D19.+ 13.46,8 v13.72,8.25 | 13.46,6.22 13.46,5.97 | 10.54,5.97 10.79,6.22 | 10.79,6.22 11.05,5.97 | 13.21,5.97 13.46,6.22 | 13.46,6.22 13.72,5.97 | 13.72,5.97 13.84,5.97 14.35,6.48 15.24,6.48 D26.+ 16.13,7.11 16.76,6.48 17.91,6.48 D33.+
PA4  (via drill 0.25)
  Top 0.203: v16.13,9.27 15.37,8.51 U2.10 | v13.46,10.92 v16.38,10.92
  Bottom 0.203: D4.+ 8.13,10.16 8.89,10.92 10.67,10.92 | D32.+ 17.91,10.92 v16.38,10.92 16.13,10.67 D25.+ v16.13,9.27 | 10.92,10.92 10.79,10.92 | 10.79,10.92 10.67,10.92 | D11.+ 10.79,10.79 | 10.79,10.79 10.79,10.92 | 10.92,10.92 10.79,10.79 | 10.79,10.79 10.67,10.92 | 10.92,10.92 v13.46,10.92 D18.+
PA5  (via drill 0.25)
  Top 0.203: U2.11 15.36,11.7 | 15.36,11.67 15.36,11.44 15.37,11.43 | v13.84,11.43 15.11,11.43 | 15.11,11.43 15.37,11.43 | 15.37,11.43 15.62,11.43 | 15.62,11.43 16,11.43 v16.13,11.56 | 15.36,11.7 15.36,11.67 | 15.36,11.67 15.11,11.43 | 15.36,11.7 15.62,11.43
  Bottom 0.203: D31.+ 17.91,13.59 16.89,13.59 16,12.7 D24.+ v16.13,11.56 | D3.+ 8.13,13.21 8.51,13.59 10.54,13.59 10.79,13.34 D10.+ 10.79,12.06 11.05,11.81 13.34,11.81 | 13.59,11.68 13.59,11.81 | 13.59,11.81 13.59,12.06 | 13.59,12.06 13.59,12.57 D17.+ | 13.72,11.56 v13.84,11.43 13.59,11.68 | 13.46,11.81 13.59,11.81 | 13.34,11.81 13.59,12.06 | 13.34,11.81 13.46,11.81 | 13.46,11.81 13.59,11.68
PA6  (via drill 0.25)
  Top 0.203: U2.12 14.71,13.56 v15.24,14.1
  VCC 0.203: v15.24,14.1 14.86,14.48 v13.97,14.48 12.19,16.26 v10.29,16.26
  Bottom 0.203: 8.13,15.49 D2.+ 8.13,14.86 8.38,14.61 10.03,14.61 D9.+ 10.79,15.49 10.29,16 v10.29,16.26 | D30.+ 17.91,16.26 16.89,16.26 16,15.37 D23.+ 16.13,14.99 v15.24,14.1 | D16.+ 13.46,14.99 v13.97,14.48
PA7  (via drill 0.25)
  Top 0.203: U2.13 14.06,13.68 v14.1,13.72
  Bottom 0.203: D1.+ 8.13,18.16 8.89,18.92 10.67,18.92 | 10.67,18.92 10.79,18.92 | 10.79,18.92 10.92,18.92 | 10.92,18.92 13.34,18.92 | 13.34,18.92 13.46,18.92 | 13.46,18.92 13.59,18.92 | 13.59,18.92 16,18.92 | 16,18.92 16.13,18.92 | 16.13,18.92 16.26,18.92 | 16.26,18.92 17.91,18.92 D29.+ | D22.+ 16.13,18.8 | 16.13,18.8 16.13,18.92 | 13.46,18.8 D15.+ 12.7,17.27 12.7,14.99 13.97,13.72 v14.1,13.72 | 13.46,18.8 13.46,18.92 | D8.+ 10.79,18.8 | 10.79,18.8 10.79,18.92 | 10.67,18.92 10.79,18.8 | 10.79,18.8 10.92,18.92 | 13.34,18.92 13.46,18.8 | 13.46,18.8 13.59,18.92 | 16,18.92 16.13,18.8 | 16.13,18.8 16.26,18.92
PB1
  Top 0.203: U2.14 13.41,11.75 13.21,11.56 11.3,11.56 9.59,9.84 R8.2
PF0  (via drill 0.25 pad 0.51)
  Top 0.203: U2.2 10.17,8.01 12.32,10.16 17.4,10.16 18.16,9.4 R9.2 18.59,8.83 v18.67,8.75
PF1
  Top 0.203: U2.3 10.82,8.03 12.57,9.78 16.64,9.78 17.14,9.27 R10.2
SWCLK/PA14  (via drill 0.25)
  Top 0.203: v9.91,16.76 9.86,16.81 8.69,16.81 7.87,16 R5.1 7.43,15.56 7.24,15.37 7.24,12.57 6.48,11.81 6.48,9.14 | 6.48,9.14 6.48,8.89 | 6.48,8.89 6.48,8.64 | v9.91,8.64 9.65,8.89 6.73,8.89 | 6.73,8.89 6.48,8.89 | 6.73,8.89 6.48,9.14 | 6.73,8.89 6.48,8.64 | 6.48,8.64 6.48,4.06 v5.84,3.43 | J7.3 12.83,2.16 v12.51,2.48
  VCC 0.203: v5.84,3.43 6.79,2.48 v12.51,2.48
  Bottom 0.203: 11.58,16.76 11.58,16.15 11.94,15.8 D16.- 11.79,15.21 11.79,13.56 11.94,13.41 D17.- | 11.58,16.76 11.58,17.42 11.56,17.45 11.94,17.83 D15.- | v9.91,16.76 11.58,16.76 | D19.- 11.94,8.64 | 11.94,8.64 D18.- | 11.94,8.64 v9.91,8.64 | D21.- 12.06,2.03 v12.51,2.48 12.32,2.67 12.32,3.56 11.94,3.94 D20.-
SWIO/PA13  (via drill 0.25)
  Top 0.203: J7.4 10.83,2.64 v11.18,2.98 | R6.1 8.89,16 9.14,16.26 v9.27,16.26
  Bottom 0.203: 9.27,17.91 D8.- v9.27,16.26 | 9.27,2.16 D14.- 9.27,2.79 | 7.37,8.51 7.37,4.3 7.72,3.94 9.27,3.94 | 7.37,8.51 7.37,8.76 | 7.37,8.76 7.37,9.02 | D13.- 9.27,3.94 | 9.27,3.94 9.27,2.79 | D10.- 9.27,11.68 8.89,11.3 7.62,11.3 | 9.27,8.76 9.02,8.76 | 9.02,8.76 7.62,8.76 | 7.62,8.76 7.37,8.76 | 9.27,8.76 9.27,9.02 | 9.27,9.02 D11.- | 7.62,8.76 7.37,9.02 | 7.62,8.76 7.37,8.51 | 9.02,8.76 9.27,9.02 | 9.02,8.76 9.27,8.51 | 9.27,15.57 D9.- v9.27,16.26 | D12.- 9.27,8.51 | 9.27,8.51 9.27,8.76 | 7.62,11.3 7.62,11.94 7.37,12.19 7.37,16 7.62,16.26 v9.27,16.26 | 7.62,11.3 7.62,10.79 7.37,10.54 7.37,9.02 | 9.27,2.79 10.99,2.79 v11.18,2.98
VIN  (via drill 0.25 pad 0.51)
  Top 0.203: 20.45,10.98 20.45,11.16 20.52,11.23
  Top 0.305: 4.95,9.14 4.95,9.27 4.51,8.83 | J1.10 4.5,8.83 | 4.51,8.83 4.9,8.83 4.95,8.89 | J2.10 20.88,11.23 | J1.2 4.5,11.23 | 4.51,11.23 4.88,11.23 4.95,11.3 | J2.10 20.52,11.23 | J2.2 20.9,8.83 | 20.88,8.83 20.52,8.83 20.45,8.76 | 4.5,11.23 4.83,11.56 | 4.5,11.23 4.51,11.23 | 4.51,11.23 4.83,10.92 | 4.5,8.83 4.51,8.83 | 4.5,8.83 4.95,8.38 | J2.10 21.71,11.23 21.72,11.24 | 20.9,8.83 20.88,8.83 | 20.88,8.83 20.57,9.14 20.57,8.51 20.9,8.83
  Top 0.406: J6.3 J6.4
  Top 0.61: J4.4 21.07,5.98 20.45,6.6 20.45,8.76 20.45,10.98 21.21,11.75 | v4.95,14.73 4.95,11.3 4.95,9.27 4.95,8.89 4.95,8.38 4.95,6.86 4.08,5.98 J6.4 | 21.21,11.75 21.53,11.43 21.46,11.43 21.21,11.68 21.21,11.75 | 21.21,11.75 21.21,14.99 | 21.21,14.99 C2.2 21.91,15.11 v22.1,15.3 | 21.21,14.99 20.51,14.99 C1.2 19.28,15.43 U1.3
  VCC 0.61: v22.1,15.3 22.03,15.3 18.41,18.92 8.13,18.92 4.95,15.75 v4.95,14.73
  Bottom 0.203: J4.3 J4.4

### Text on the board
tPlace: 6 | 6 | 5 | 5 | 4 | 4 | 3 | 3 | 2 | 2 | 1 | !RST | SWIO | SCLK | GND | 3V3 | 1
bPlace: GND | GND | INT2 | INT2 | INT1 | INT1 | v1.0 | 10/14/2015 | VCC | VCC | SCL | Xadow LED 5x7 | SCL | SDA | SDA

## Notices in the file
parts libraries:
moudle-new: This work is licensed under the Creative Commons Attribution 4.0 International License.
To view a copy of this license,visit:
http://creativecommons.org/licenses/by-sa/4.0
moudle-new: CC-BY-SA
